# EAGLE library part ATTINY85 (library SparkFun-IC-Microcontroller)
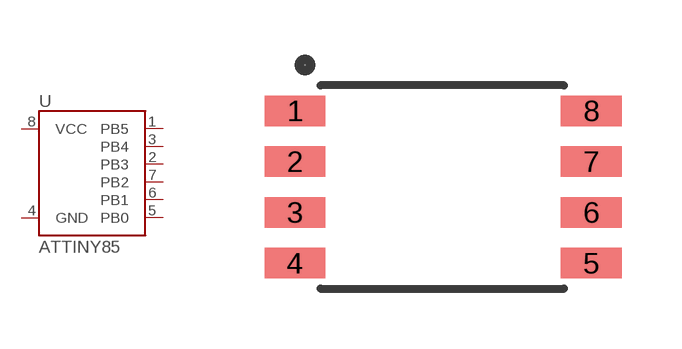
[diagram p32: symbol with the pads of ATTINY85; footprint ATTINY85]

Designator prefix U

## ATTINY85 (PROD_ID: IC-09092)  [ATTINY85]
1  PB5
2  PB3
3  PB4
4  GND
5  PB0
6  PB1
7  PB2
8  VCC

## Footprint ATTINY85 (pad centres in mm)
smd 1.524 x 0.762: 1 -3.683,1.905; 2 -3.683,0.635; 3 -3.683,-0.635; 4 -3.683,-1.905; 5 3.727,-1.905; 6 3.727,-0.635; 7 3.727,0.635; 8 3.727,1.905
